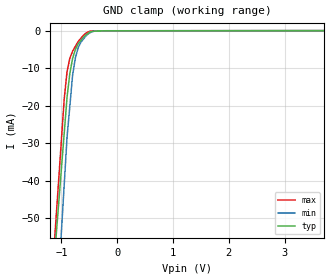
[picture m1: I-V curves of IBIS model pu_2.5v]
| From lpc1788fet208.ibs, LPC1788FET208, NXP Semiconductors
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[Model] pu_2.5v
Model_type Input
Vinl = 750.000mV
Vinh = 1.75000V
C_comp 900.000fF 855.000fF 945.000fF
| variable typ   min   max
[Voltage Range] 2.50000V 2.40000V 2.60000V
[POWER Clamp Reference] 2.50000V 2.40000V 2.60000V
[GND Clamp Reference] 0.00000V 0.00000V 0.00000V
[Temperature Range]   25   85   -40
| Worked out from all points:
|   GND clamp passes 1 mA (typ) near -0.55 V on its own axis
[GND Clamp]
-2.5V     -320.9mA   -428.2mA   -355.8mA
-950mV    -27.31mA   -41.03mA   -18.18mA
-900mV    -17.84mA   -28.54mA   -11.01mA
-850mV    -11.49mA   -20.22mA   -7.415mA
-800mV    -7.413mA   -11.9mA    -5.476mA
-750mV    -5.014mA   -7.253mA   -4.181mA
-700mV    -3.535mA   -4.543mA   -2.887mA
-650mV    -2.594mA   -3.07mA    -2.015mA
-550mV    -1.057mA   -1.212mA   -539.5uA
-400mV    -147.5uA   -112.4uA   -63.11uA
-200mV    -36.9uA    -30.37uA   -38.72uA
5V        16.89uA    16.03uA    16.38uA
[POWER Clamp]
-2.5V     0A         0A         0A
5V        0A         0A         0A
